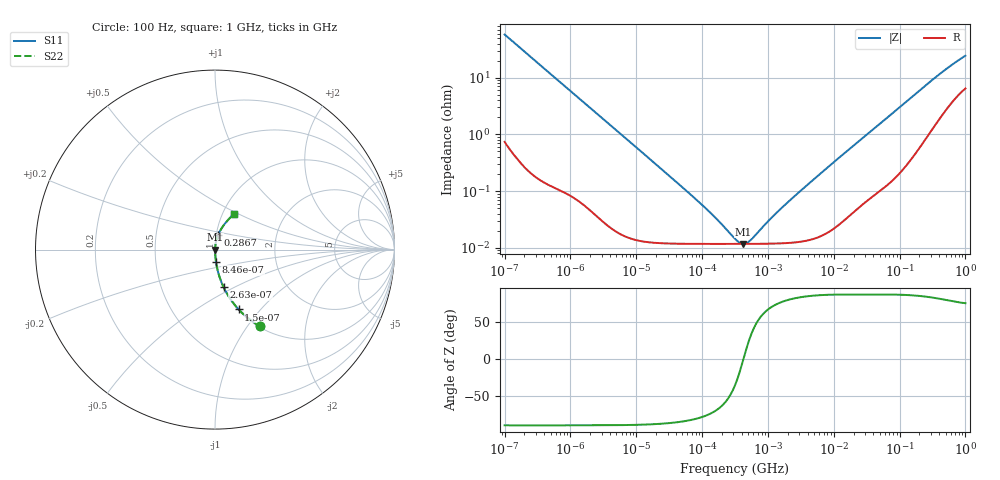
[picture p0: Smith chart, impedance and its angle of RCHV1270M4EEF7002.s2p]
! RCHV1270M4EEF7002  S-PARAMETER MODEL  (AEC-Q200 qualified)
! Model Generated by ELNA Corporation (http://www.ty-top.com)
! Version 1.0
! ELNA Control No. 240229
! Copyright (c) 2024 ELNA CO.,LTD. All Rights Reserved.
! Products Name : CONDUCTIVE POLYMER HYBRID ALUMINUM ELECTROLYTIC CAPACITORS
! Characteristics :
!  Capacitance  :  27uF  ,  Rated voltage  :  63V
!  Operating Temp. Range  :  -55 to +105 degC  ,  Endurance  :  5000hr at 105 degC
!  Dimension D  :  8mm  ,  Dimension L  :  8.7mm
! Frequency Range : 100Hz - 1GHz
! External Node Assignments :
!  1  o---| |---o  2
# MHz S RI R 50
!Freq[MHz].  S11 Real  S11 Imag  S21 Real  S21 Imag  S12 Real  S12 Imag  S22 Real  S22 Imag
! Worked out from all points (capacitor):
!   401 points, 100 Hz to 1 GHz, reference 50 ohm
!   read as one part in series: C = 27.6 uF near 108 Hz
!   lowest |Z| = 11.7 mohm at 419.3 kHz (marker M1)
!   series resonance near 425.8 kHz, so ESL is about 5.1 nH
!   S11 on the Smith chart (normalised r, x): 100 Hz: 1.01, -1.15; 150 Hz: 1.01, -0.77; 263 Hz: 1.00, -0.44; 846 Hz: 1.00, -0.14; 286.7 MHz: 1.02, +0.17; 1 GHz: 1.13, +0.47
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0.0001  0.2528 -0.4283  0.7472 0.4283  0.7472 0.4283  0.2528 -0.4283
0.00015  0.1322 -0.3337  0.8678 0.3337  0.8678 0.3337  0.1322 -0.3337
0.000198  0.0802 -0.2671  0.9198 0.2671  0.9198 0.2671  0.0802 -0.2671
0.000263  0.0477 -0.2088  0.9523 0.2088  0.9523 0.2088  0.0477 -0.2088
0.000462  0.0167 -0.1229  0.9833 0.1229  0.9833 0.1229  0.0167 -0.1229
0.000846  0.0056 -0.0682  0.9944 0.0682  0.9944 0.0682  0.0056 -0.0682
0.001488  0.00214 -0.0392  0.9979 0.0392  0.9979 0.0392  0.00214 -0.0392
0.004241  0.00041 -0.0139  0.9996 0.0139  0.9996 0.0139  0.00041 -0.0139
0.022131  0.000128 -0.00266  0.9999 0.00266  0.9999 0.00266  0.000128 -0.00266
0.115478  0.000117 -0.000474  0.9999 0.000474  0.9999 0.000474  0.000117 -0.000474
0.179887  0.000117 -0.00027  0.9999 0.00027  0.9999 0.00027  0.000117 -0.00027
0.316228  0.000117 -8.38e-05  0.9999 8.38e-05  0.9999 8.38e-05  0.000117 -8.38e-05
0.371535  0.000117 -3.79e-05  0.9999 3.79e-05  0.9999 3.79e-05  0.000117 -3.79e-05
0.419276  0.000117 -4.26e-06  0.9999 4.26e-06  0.9999 4.26e-06  0.000117 -4.26e-06
0.473151  0.000117 2.93e-05  0.9999 -2.93e-05  0.9999 -2.93e-05  0.000117 2.93e-05
0.555904  0.000117 7.49e-05  0.9999 -7.49e-05  0.9999 -7.49e-05  0.000117 7.49e-05
1.348963  0.000119 0.000396  0.9999 -0.000396  0.9999 -0.000396  0.000119 0.000396
4.704354  0.000143 0.00152  0.9999 -0.00152  0.9999 -0.00152  0.000143 0.00152
69.9842  0.00181 0.0211  0.9982 -0.0211  0.9982 -0.0211  0.00181 0.0211
286.7477  0.0171 0.0808  0.9829 -0.0808  0.9829 -0.0808  0.0171 0.0808
568.8529  0.0517 0.1402  0.9483 -0.1402  0.9483 -0.1402  0.0517 0.1402
1000  0.1044 0.1982  0.8956 -0.1982  0.8956 -0.1982  0.1044 0.1982
